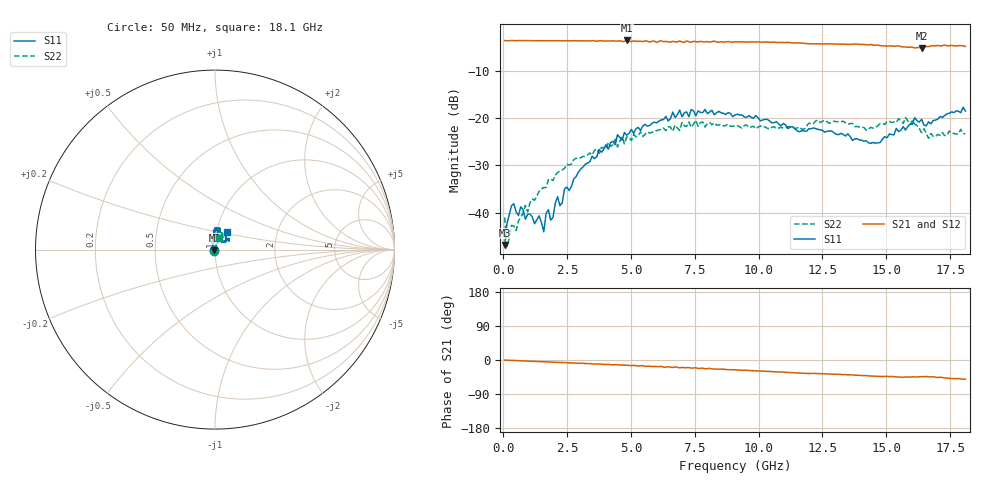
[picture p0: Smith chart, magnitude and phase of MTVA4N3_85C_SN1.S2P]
! Network Analyzer HP8720D.06.14 Serial No. US36140669
! 11 May 2005  10:08:16
! Frequency  S11  S21  S12  S22
# HZ  S  DB R 50
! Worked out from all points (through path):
!   201 points, 50 MHz to 18.1 GHz, reference 50 ohm
!   highest |S21| = -3.59 dB at 4.833 GHz (marker M1); lowest = -5.2 dB at 16.39 GHz (marker M2)
!   group delay of S21, straight-line fit = 7.79 ps
!   lowest |S11| = -46.9 dB at 50 MHz (marker M3), VSWR 1.01, Z = 49.7 - j0.299 ohm
!   |S11| at or under -10 dB: start of sweep to end of sweep
!   |S22| runs from -47.1 to -19.9 dB; largest |S21 - S12| = 0.025
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5e7  -46.87 -138.4  -3.61 -0.3  -3.63 -0.6  -41.04 -142.8
1.4025e8  -42.39 -158.0  -3.66 -0.5  -3.65 -0.9  -47.12 -169.1
3.2075e8  -38.57 -175.4  -3.61 -0.9  -3.62 -1.3  -42.71 -170.8
5.0125e8  -39.87 -165.4  -3.64 -1.6  -3.62 -2.0  -43.81 155.4
8.6225e8  -41.41 169.7  -3.62 -2.5  -3.63 -2.9  -38.47 148.0
1.40375e9  -40.70 145.2  -3.63 -4.2  -3.64 -4.5  -35.49 128.6
1.58425e9  -44.08 121.2  -3.64 -4.7  -3.64 -5.0  -34.71 120.8
1.6745e9  -40.20 108.3  -3.64 -4.9  -3.64 -5.3  -34.70 121.4
1.94525e9  -41.05 92.5  -3.66 -5.6  -3.66 -6.1  -33.23 112.9
2.12575e9  -36.65 97.6  -3.64 -6.2  -3.65 -6.5  -31.54 110.8
2.216e9  -38.53 97.3  -3.65 -6.5  -3.63 -6.8  -31.18 107.5
3.1185e9  -30.39 72.9  -3.67 -8.8  -3.68 -9.4  -28.14 118.3
4.83325e9  -23.63 78.1  -3.59 -13.7  -3.67 -14.8  -24.03 91.8
6.09675e9  -20.65 77.6  -3.76 -17.6  -3.69 -17.9  -22.57 85.3
6.909e9  -18.33 79.2  -3.69 -20.5  -3.80 -20.0  -22.66 78.0
9.075e9  -19.37 89.6  -3.89 -26.0  -3.85 -26.4  -21.57 69.8
1.21435e10  -22.09 91.8  -4.31 -35.2  -4.27 -35.7  -21.21 77.9
1.439975e10  -25.36 47.8  -4.46 -42.3  -4.44 -42.6  -21.96 76.9
1.512175e10  -23.40 42.5  -4.78 -43.9  -4.65 -43.9  -20.70 77.4
1.57535e10  -22.57 41.5  -4.95 -44.7  -5.09 -45.9  -19.89 67.0
1.638525e10  -20.28 34.9  -5.18 -43.9  -5.01 -43.9  -23.11 59.2
1.81e10  -18.54 54.7  -4.86 -50.4  -4.89 -51.6  -23.35 73.1
